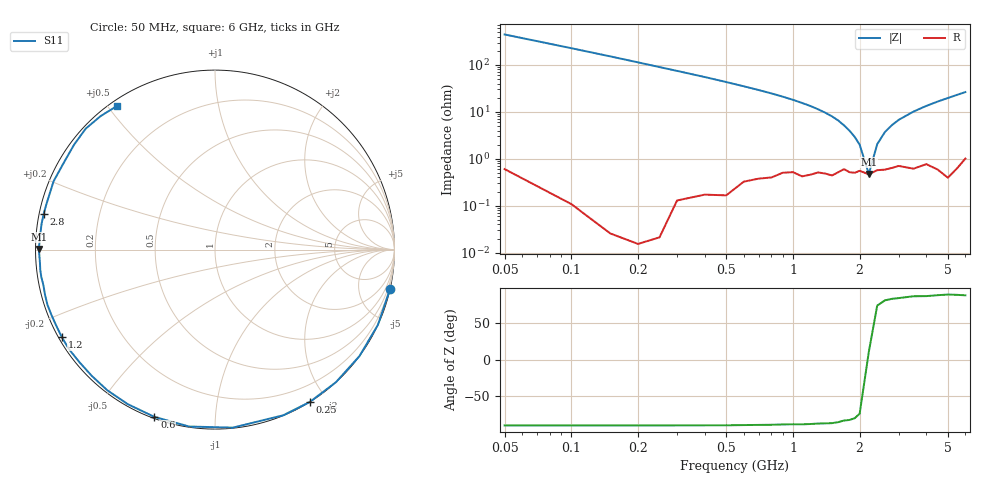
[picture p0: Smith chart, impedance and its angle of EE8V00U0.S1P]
! Infineon Technologies  Discrete & RF Semiconductors
! BBY55-02W
! Si Tuning Diode in SCD-80
! VR = 8 V
! S-Parameters:  June  2000
# GHz  S  MA  R  50
!  f  S11
! GHz  MAG  ANG
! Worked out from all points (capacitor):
!   34 points, 50 MHz to 6 GHz, reference 50 ohm
!   read as one part to ground: C = 6.98 pF near 50 MHz
!   lowest |Z| = 475 mohm at 2.2 GHz (marker M1)
!   series resonance near 2.191 GHz, so ESL is about 760 pH
!   S11 on the Smith chart (normalised r, x): 50 MHz: 0.01, -8.92; 250 MHz: 0.00, -1.80; 600 MHz: 0.01, -0.70; 1.2 GHz: 0.01, -0.27; 2.8 GHz: 0.01, +0.10; 6 GHz: 0.02, +0.53
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0.05  0.9997 -12.8
0.1  0.9998 -24.8
0.15  0.9999 -36.4
0.2  0.9999 -47.6
0.25  0.9998 -58.1
0.3  0.9984 -67.6
0.4  0.9969 -84.3
0.5  0.9962 -98.3
0.6  0.9913 -109.9
0.7  0.9888 -119.4
0.8  0.9872 -127.4
0.9  0.983 -134.3
1  0.9818 -140.3
1.1  0.9847 -145.6
1.2  0.983 -150.2
1.4  0.9815 -158.3
1.6  0.9799 -165.1
1.7  0.9764 -168.3
1.8  0.9796 -171.0
2.2  0.9815 179.8
2.4  0.9774 175.5
2.8  0.975 168.1
3.5  0.9766 157.1
4  0.9717 150.0
4.5  0.979 143.3
5  0.9864 136.9
5.5  0.9796 130.6
6  0.9689 124.3
